PROGRAM MAIN
VAR
	byByte		AT %MB0 : ARRAY [0..1027] OF BYTE;
	i			: INT;
	moreBytes	: ARRAY [0..8192] OF BYTE;
	bInitTest: BOOL := FALSE;
	bStartTest: BOOL := FALSE;
	bTestBusy: BOOL := FALSE;
	nTestState: DINT := 0;
	nTestCasesFailed: DINT := 0;
	sLogPath: T_MaxString := 'var/log';
END_VAR

FOR i := 4 TO 1027 BY 1 DO
	byByte[i] := byByte[i] + 1;
END_FOR

END_PROGRAM
